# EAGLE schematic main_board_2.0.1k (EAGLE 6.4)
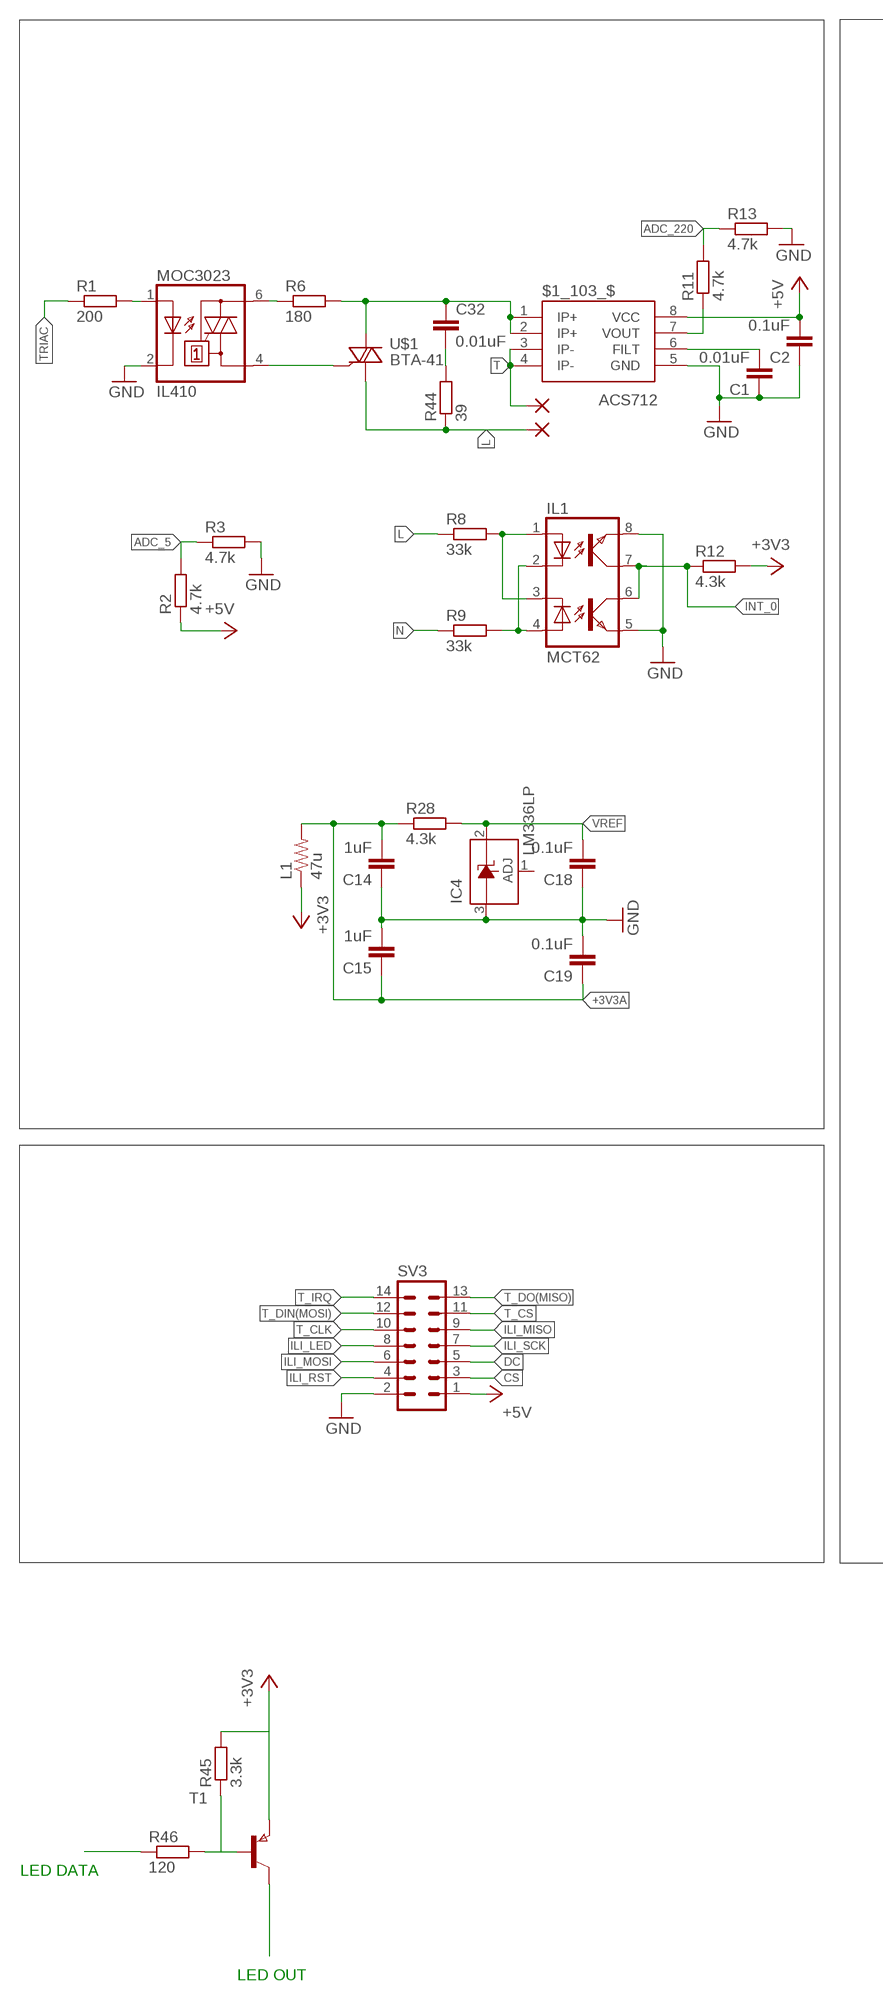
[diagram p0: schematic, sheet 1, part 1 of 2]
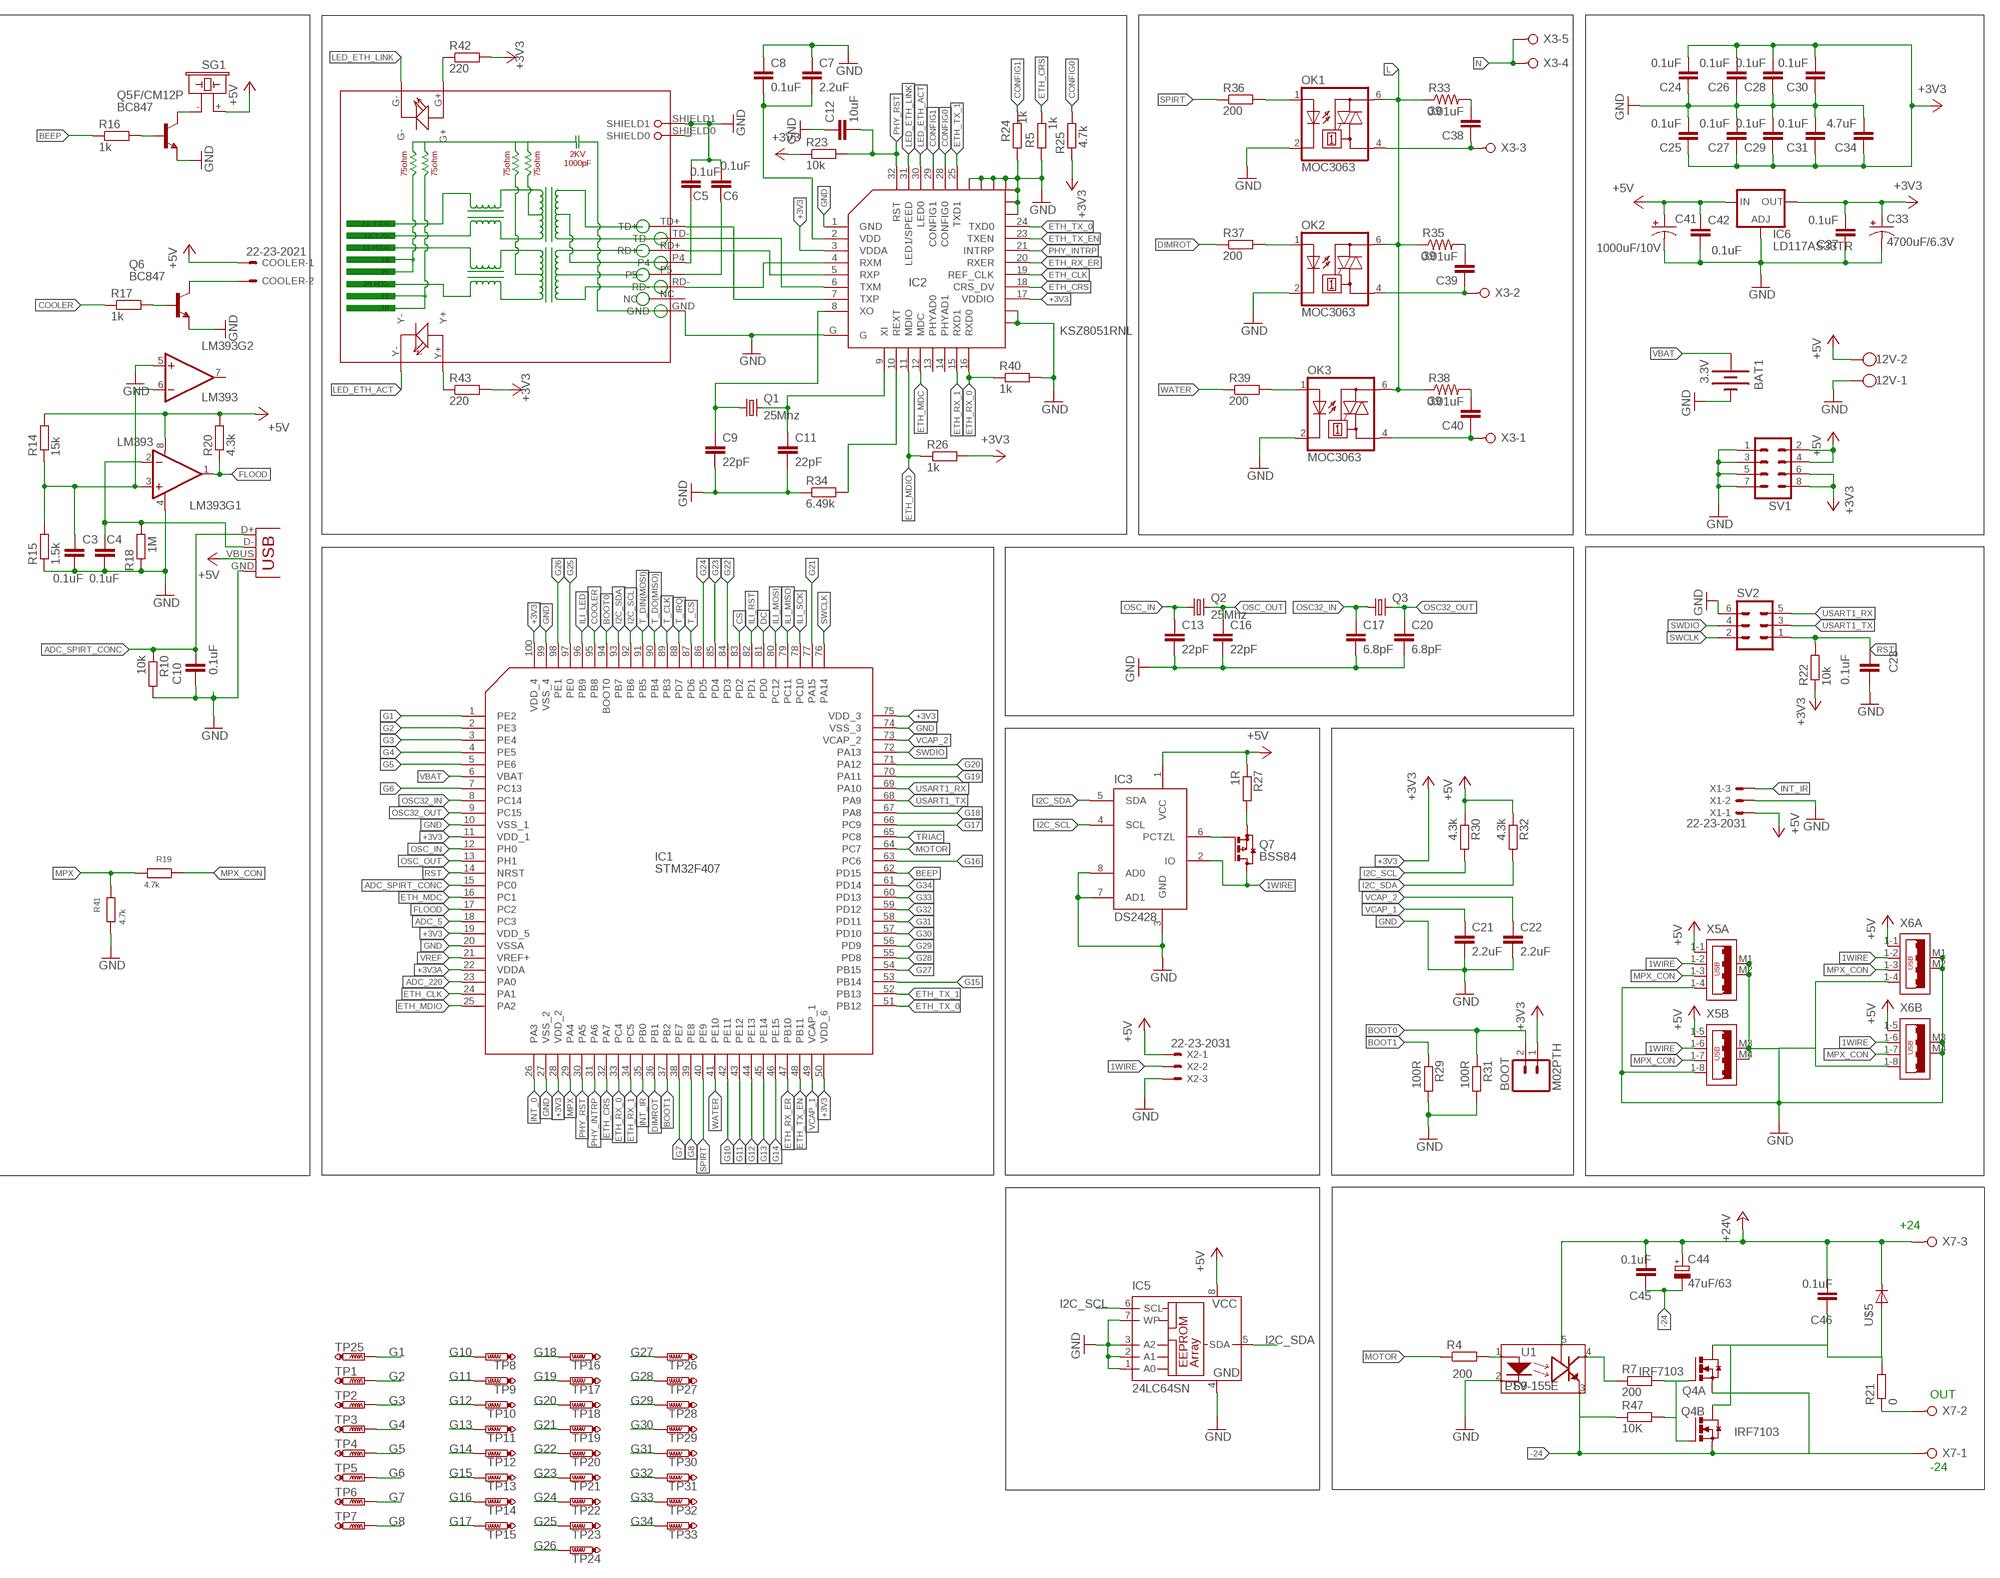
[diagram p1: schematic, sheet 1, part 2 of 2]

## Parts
12V  W237-102  [W237-102]
$1_103_$  ACS712  [SO08]
BAT1  3.3V  BATTERY20PTH  [BATTCOM_20MM_PTH]
BOOT  M02PTH  [1X02]
C1  0.01uF  C-EUC0603  [C0603]
C2  0.1uF  C-EUC0603  [C0603]
C3  0.1uF  C-EUC0603  [C0603]
C4  0.1uF  C-EUC0603  [C0603]
C5  0.1uF  C-EUC0603  [C0603]
C6  0.1uF  C-EUC0603  [C0603]
C7  2.2uF  C-EUC0603  [C0603]
C8  0.1uF  C-EUC0603  [C0603]
C9  22pF  C-EUC0603  [C0603]
C10  0.1uF  C-EUC0603  [C0603]
C11  22pF  C-EUC0603  [C0603]
C12  10uF  CAP1206  [1206]
C13  22pF  C-EUC0603  [C0603]
C14  1uF  C-EUC0603  [C0603]
C15  1uF  C-EUC0603  [C0603]
C16  22pF  C-EUC0603  [C0603]
C17  6.8pF  C-EUC0603  [C0603]
C18  0.1uF  C-EUC0603  [C0603]
C19  0.1uF  C-EUC0603  [C0603]
C20  6.8pF  C-EUC0603  [C0603]
C21  2.2uF  C-EUC0603  [C0603]
C22  2.2uF  C-EUC0603  [C0603]
C23  0.1uF  C-EUC0603  [C0603]
C24  0.1uF  C-EUC0603  [C0603]
C25  0.1uF  C-EUC0603  [C0603]
C26  0.1uF  C-EUC0603  [C0603]
C27  0.1uF  C-EUC0603  [C0603]
C28  0.1uF  C-EUC0603  [C0603]
C29  0.1uF  C-EUC0603  [C0603]
C30  0.1uF  C-EUC0603  [C0603]
C31  0.1uF  C-EUC0603  [C0603]
C32  0.01uF  C-EU075-032X103  [C075-032X103]
C33  4700uF/6.3V  CPOL-USE5-13  [E5-13]
C34  4.7uF  C-EUC0603  [C0603]
C37  0.1uF  C-EUC0603  [C0603]
C38  0.01uF  CAPPTH3  [CAP-PTH-LARGE]
C39  0.01uF  CAPPTH3  [CAP-PTH-LARGE]
C40  0.01uF  CAPPTH3  [CAP-PTH-LARGE]
C41  1000uF/10V  CPOL-USE5-8.5  [E5-8,5]
C42  0.1uF  C-EUC0603  [C0603]
C44  47uF/63  CPOL-EUE5-10.5  [E5-10,5]
C45  0.1uF  C-EUC0603  [C0603]
C46  0.1uF  C-EUC0603  [C0603]
COOLER  22-23-2021  [22-23-2021]
IC1  STM32F407  [LQFP100]
IC2  KSZ8051RNL  [QFN32]
IC3  DS2428  [SO08]
IC4  LM336LP  [TO92]
IC5  24LC64SN  [SO-08]
IC6  LD117AS33TR  [SOT223]
IL1  MCT62  [DIL8]
JP1  USB-B  USBPTH  [USB-B-PTH]
L  PAD-220  [PAD-220]
L1  47u  RESISTOR2010  [R2010]
LM393  LM393  [SO08]
MOC3023  IL410  [DIL06]
OK1  MOC3063  MOC3023M  [DIL06]
OK2  MOC3063  MOC3023M  [DIL06]
OK3  MOC3063  MOC3023M  [DIL06]
Q1  25Mhz  CRYSTALHC49U-V  [HC49U-V]
Q2  25Mhz  CRYSTALHC49U-V  [HC49U-V]
Q3  CRYSTALTC38H  [TC38H]
Q4  IRF7103  IRF8313P  [SO-08]
Q5  BC847  [SOT23]
Q6  BC847  [SOT23]
Q7  BSS84  [SOT23]
R1  200  R-EU_R0603  [R0603]
R2  4.7k  R-EU_R0603  [R0603]
R3  4.7k  R-EU_R0603  [R0603]
R4  200  R-EU_R0603  [R0603]
R5  1k  R-EU_R0603  [R0603]
R6  180  R-EU_0204/2V  [0204V]
R7  200  R-EU_R0603  [R0603]
R8  33k  R-EU_0617/5V  [0617V]
R9  33k  R-EU_0617/5V  [0617V]
R10  10k  R-EU_R0603  [R0603]
R11  4.7k  R-EU_R0603  [R0603]
R12  4.3k  R-EU_R0603  [R0603]
R13  4.7k  R-EU_R0603  [R0603]
R14  15k  R-EU_R0603  [R0603]
R15  1.5k  R-EU_R0603  [R0603]
R16  1k  R-EU_R0603  [R0603]
R17  1k  R-EU_R0603  [R0603]
R18  1M  R-EU_R0603  [R0603]
R19  4.7k  R-EU_R0603  [R0603]
R20  4.3k  R-EU_R0603  [R0603]
R21  0  R-EU_R1206  [R1206]
R22  10k  R-EU_R0603  [R0603]
R23  10k  R-EU_R0603  [R0603]
R24  1k  R-EU_R0603  [R0603]
R25  4.7k  R-EU_R0603  [R0603]
R26  1k  R-EU_R0603  [R0603]
R27  1R  R-EU_R0603  [R0603]
R28  4.3k  R-EU_R0603  [R0603]
R29  100R  R-EU_R0603  [R0603]
R30  4.3k  R-EU_R0603  [R0603]
R31  100R  R-EU_R0603  [R0603]
R32  4.3k  R-EU_R0603  [R0603]
R33  39  RESISTOR2512  [R2512]
R34  6.49k  R-EU_R0805  [R0805]
R35  39  RESISTOR2512  [R2512]
R36  200  R-EU_R0603  [R0603]
R37  200  R-EU_R0603  [R0603]
R38  39  RESISTOR2512  [R2512]
R39  200  R-EU_R0603  [R0603]
R40  1k  R-EU_R0603  [R0603]
R41  4.7k  R-EU_R0603  [R0603]
R42  220  R-EU_R0603  [R0603]
R43  220  R-EU_R0603  [R0603]
R44  39  R-EU_0613/5V  [P0613V]
R45  3.3k  R-EU_R0603  [R0603]
R46  120  R-EU_R0603  [R0603]
R47  10K  R-EU_R0603  [R0603]
RJ1  HR911105A  [HR911105A]
SG1  F/CM12P  [F/CM12P]
SV1  MA04-2  [MA04-2]
SV2  MA03-2  [MA03-2]
SV3  ML14  [ML14]
T  PAD-220  [PAD-220]
T1  PNPSOT23  [SOT-23]
TP1  PTR1MY0012X0024  [MY]
TP2  PTR1MY0012X0024  [MY]
TP3  PTR1MY0012X0024  [MY]
TP4  PTR1MY0012X0024  [MY]
TP5  PTR1MY0012X0024  [MY]
TP6  PTR1MY0012X0024  [MY]
TP7  PTR1MY0012X0024  [MY]
TP8  PTR1MY0012X0024  [MY]
TP9  PTR1MY0012X0024  [MY]
TP10  PTR1MY0012X0024  [MY]
TP11  PTR1MY0012X0024  [MY]
TP12  PTR1MY0012X0024  [MY]
TP13  PTR1MY0012X0024  [MY]
TP14  PTR1MY0012X0024  [MY]
TP15  PTR1MY0012X0024  [MY]
TP16  PTR1MY0012X0024  [MY]
TP17  PTR1MY0012X0024  [MY]
TP18  PTR1MY0012X0024  [MY]
TP19  PTR1MY0012X0024  [MY]
TP20  PTR1MY0012X0024  [MY]
TP21  PTR1MY0012X0024  [MY]
TP22  PTR1MY0012X0024  [MY]
TP23  PTR1MY0012X0024  [MY]
TP24  PTR1MY0012X0024  [MY]
TP25  PTR1MY0012X0024  [MY]
TP26  PTR1MY0012X0024  [MY]
TP27  PTR1MY0012X0024  [MY]
TP28  PTR1MY0012X0024  [MY]
TP29  PTR1MY0012X0024  [MY]
TP30  PTR1MY0012X0024  [MY]
TP31  PTR1MY0012X0024  [MY]
TP32  PTR1MY0012X0024  [MY]
TP33  PTR1MY0012X0024  [MY]
U1  LTV-155E  OPTO:PS9__  [PANASONIC_SOP5]
U$1  BTA-41  [TOP3L]
U$5  DIODE-SMB  [SMB]
X1  22-23-2031  [22-23-2031]
X2  22-23-2031  [22-23-2031]
X3  W237-05P  [W237-5P]
X5  USB_3PSHIELD-85-32003-00X-1  [85-32003-00X-1]
X6  USB_3PSHIELD-85-32003-00X-1  [85-32003-00X-1]
X7  W237-03P  [W237-133]

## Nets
1WIRE: IC3.2(IO) Q7.3(D) X2.2 X5.1-2 X5.1-6 X6.1-2 X6.1-6
+3V3 [+3V3]: BOOT.1 C24.2 C25.1 C26.2 C27.1 C28.2 C29.1 C30.2 C31.1 C33.+ C34.1 C37.2 IC1.11(VDD_1) IC1.19(VDD_5) IC1.28(VDD_2) IC1.50(VDD_6) IC1.75(VDD_3) IC1.100(VDD_4) IC2.3(VDDA) IC2.17(VDDIO) IC6.4(OUT) L1.1 R12.2 R22.1 R23.1 R25.1 R26.2 R42.2 R43.2 R45.2 SV1.6 SV1.8 T1.2(E)
+3V3A: C14.2 C15.1 C19.1 IC1.22(VDDA) L1.2 R28.1
+5V [+5V]: 12V.2 $1_103_$.8(VCC) C2.2 C41.+ C42.2 COOLER.1 IC3.1(VCC) IC5.8(VCC) IC6.3(IN) JP1.VBUS LM393.8(V+) R2.1 R14.2 R20.2 R27.1 R30.1 R32.1 SG1.+ SV1.2 SV1.4 SV3.1 X1.1 X2.1 X5.1-1 X5.1-5 X6.1-1 X6.1-5
+24V: C44.+ C45.2 C46.2 U1.5(VCC) U$5.C X7.3
-24: C44.- C45.1 Q4.1(B:S) Q4.3(A:S) R47.1 U1.3(COM) X7.1
ADC_5: IC1.18(PC3) R2.2 R3.1
ADC_220: IC1.23(PA0) R11.2 R13.1
ADC_SPIRT_CONC: C10.2 IC1.15(PC0) JP1.D+ R10.1
BEEP: IC1.62(PD15) R16.1
BOOT0: BOOT.2 IC1.94(BOOT0) R31.1
BOOT1: IC1.37(PB2) R29.1
CONFIG0: IC2.28(CONFIG0) R25.2
CONFIG1: IC2.29(CONFIG1) R24.2
COOLER: IC1.95(PB8) R17.1
CS: IC1.83(PD2) SV3.3
DC: IC1.81(PD0) SV3.5
DIMROT: IC1.36(PB1) R37.1
DRAIN: C46.1 Q4.5(A:D) Q4.6(A:D) Q4.7(B:D) Q4.8(B:D) R21.2 U$5.A
ETH_CLK: IC1.24(PA1) IC2.19(REF_CLK)
ETH_CRS: IC1.32(PA7) IC2.18(CRS_DV) R5.2
ETH_MDC: IC1.16(PC1) IC2.12(MDC)
ETH_MDIO: IC1.25(PA2) IC2.11(MDIO) R26.1
ETH_RX_0: IC1.33(PC4) IC2.16(RXD0) R40.1
ETH_RX_1: IC1.34(PC5) IC2.15(RXD1)
ETH_RX_ER: IC1.47(PB10) IC2.20(RXER)
ETH_TX_0: IC1.51(PB12) IC2.24(TXD0)
ETH_TX_1: IC1.52(PB13) IC2.25(TXD1)
ETH_TX_EN: IC1.48(PB11) IC2.23(TXEN)
FLOOD: IC1.17(PC2) LM393.1(OUT) R20.1
G1: IC1.1(PE2) TP25.P$1(TP)
G2: IC1.2(PE3) TP1.P$1(TP)
G3: IC1.3(PE4) TP2.P$1(TP)
G4: IC1.4(PE5) TP3.P$1(TP)
G5: IC1.5(PE6) TP4.P$1(TP)
G6: IC1.7(PC13) TP5.P$1(TP)
G7: IC1.38(PE7) TP6.P$1(TP)
G8: IC1.39(PE8) TP7.P$1(TP)
G10: IC1.42(PE11) TP8.P$1(TP)
G11: IC1.43(PE12) TP9.P$1(TP)
G12: IC1.44(PE13) TP10.P$1(TP)
G13: IC1.45(PE14) TP11.P$1(TP)
G14: IC1.46(PE15) TP12.P$1(TP)
G15: IC1.53(PB14) TP13.P$1(TP)
G16: IC1.63(PC6) TP14.P$1(TP)
G17: IC1.66(PC9) TP15.P$1(TP)
G18: IC1.67(PA8) TP16.P$1(TP)
G19: IC1.70(PA11) TP17.P$1(TP)
G20: IC1.71(PA12) TP18.P$1(TP)
G21: IC1.77(PA15) TP19.P$1(TP)
G22: IC1.84(PD3) TP20.P$1(TP)
G23: IC1.85(PD4) TP21.P$1(TP)
G24: IC1.86(PD5) TP22.P$1(TP)
G25: IC1.97(PE0) TP23.P$1(TP)
G26: IC1.98(PE1) TP24.P$1(TP)
G27: IC1.54(PB15) TP26.P$1(TP)
G28: IC1.55(PD8) TP27.P$1(TP)
G29: IC1.56(PD9) TP28.P$1(TP)
G30: IC1.57(PD10) TP29.P$1(TP)
G31: IC1.58(PD11) TP30.P$1(TP)
G32: IC1.59(PD12) TP31.P$1(TP)
G33: IC1.60(PD13) TP32.P$1(TP)
G34: IC1.61(PD14) TP33.P$1(TP)
GND: 12V.1 $1_103_$.5(GND) BAT1.2(-) C1.1 C2.1 C3.1 C4.1 C5.2 C6.2 C7.1 C8.1 C9.2 C10.1 C11.2 C12.1 C13.2 C14.1 C15.2 C16.2 C17.2 C18.1 C19.2 C20.2 C21.2 C22.2 C23.2 C24.1 C25.2 C26.1 C27.2 C28.1 C29.2 C30.1 C31.2 C33.- C34.2 C37.1 C41.- C42.1 IC1.10(VSS_1) IC1.20(VSSA) IC1.27(VSS_2) IC1.74(VSS_3) IC1.99(VSS_4) IC2.1(GND) IC2.G IC2.P$2(GND1) IC2.P$3(GND2) IC2.P$4(GND3) IC2.P$5(GND4) IC2.P$6(GND5) IC2.P$7(GND6) IC2.P$8(GND7) IC2.P$9(GND8) IC2.P$10(GND9) IC3.3(GND) IC3.7(AD1) IC3.8(AD0) IC4.3(A) IC5.1(A0) IC5.2(A1) IC5.3(A2) IC5.4(GND) IC5.7(WP) IC6.1(ADJ) IL1.5(EMIT1) IL1.8(EMIT) JP1.GND LM393.4(V-) LM393.5(+IN) MOC3023.2(C) OK1.2(C) OK2.2(C) OK3.2(C) Q5.2(E) Q6.2(E) R3.2 R5.1 R10.2 R13.2 R15.1 R18.1 R24.1 R29.2 R31.2 R34.1 R40.2 R41.2 RJ1.GND RJ1.SHIELD0 RJ1.SHIELD1 SV1.1 SV1.3 SV1.5 SV1.7 SV2.6 SV3.2 U1.2(K) X1.2 X2.3 X5.1-4 X5.1-8 X5.M1(A:M6) X5.M2(A:M7) X5.M3(B:M6) X5.M4(B:M7) X6.1-4 X6.1-8 X6.M1(A:M6) X6.M2(A:M7) X6.M3(B:M6) X6.M4(B:M7)
I2C_SCL: IC1.92(PB6) IC3.4(SCL) IC5.6(SCL) R30.2
I2C_SDA: IC1.93(PB7) IC3.5(SDA) IC5.5(SDA) R32.2
ILI_LED: IC1.96(PB9) SV3.8
ILI_MISO: IC1.79(PC11) SV3.9
ILI_MOSI: IC1.80(PC12) SV3.6
ILI_RST: IC1.82(PD1) SV3.4
ILI_SCK: IC1.78(PC10) SV3.7
INT_0: IC1.26(PA3) IL1.6(COL1) IL1.7(COL) R12.1
INT_IR: IC1.35(PB0) X1.3
L: L.1(P) OK1.6(A2) OK2.6(A2) OK3.6(A2) R8.1 R33.1 R35.1 R38.1 R44.1 U$1.A1
LED_ETH_ACT: IC2.30(LED0) RJ1.Y-
LED_ETH_LINK: IC2.31(LED1/SPEED) RJ1.G-
LT: $1_103_$.1(IP+) $1_103_$.2(IP+) C32.1 R6.2 U$1.A2
MOTOR: IC1.64(PC7) R4.1
MPX: IC1.29(PA4) R19.2 R41.1
MPX_CON: R19.1 X5.1-3 X5.1-7 X6.1-3 X6.1-7
N: R9.1 X3.4 X3.5
N$1: IC3.6(PCTZL) Q7.1(G)
N$2: Q5.3(C) SG1.-
N$3: Q5.1(B) R16.2
N$4: COOLER.2 Q6.3(C)
N$5: Q6.1(B) R17.2
N$6: IC2.10(REXT) R34.2
N$7: R4.2 U1.1(A)
N$8: C7.2 C8.2 IC2.2(VDD)
N$9: C9.1 IC2.8(XO) Q1.1
N$10: C11.1 IC2.9(XI) Q1.2
N$11: IC2.5(RXP) RJ1.RD+
N$12: IC2.6(TXM) RJ1.TD-
N$13: IC2.7(TXP) RJ1.TD+
N$14: C5.1 RJ1.P4
N$15: IC2.4(RXM) RJ1.RD-
N$16: C6.1 RJ1.P5
N$17: IL1.1(A) IL1.3(C1) R8.2
N$18: Q4.2(B:G) Q4.4(A:G) R7.2 R47.2
N$19: T1.1(C)
N$21: C32.2 R44.2
N$22: R42.1 RJ1.G+
N$23: C3.2 LM393.3(+IN) LM393.6(-IN) R14.1 R15.2
N$24: C4.2 JP1.D- LM393.2(-IN) R18.2
N$26: Q7.2(S) R27.2
N$27: R45.1 R46.2 T1.3(B)
N$28: R7.1 U1.4(OC)
N$29: OK1.1(A) R36.2
N$30: OK2.1(A) R37.2
N$31: MOC3023.6(A2) R6.1
N$32: $1_103_$.7(VOUT) R11.1
N$33: IL1.2(C) IL1.4(A1) R9.2
N$34: C39.2 R35.2
N$35: MOC3023.1(A) R1.2
N$36: $1_103_$.6(FILT) C1.2
N$37: C38.2 R33.2
N$38: R21.1 X7.2
N$39: R43.1 RJ1.Y+
N$40: R46.1
N$42: C38.1 OK1.4(A1) X3.3
N$43: C39.1 OK2.4(A1) X3.2
N$44: OK3.1(A) R39.2
N$45: C40.2 R38.2
N$48: C40.1 OK3.4(A1) X3.1
OSC32_IN: C17.1 IC1.8(PC14) Q3.1
OSC32_OUT: C20.1 IC1.9(PC15) Q3.2
OSC_IN: C13.1 IC1.12(PH0) Q2.1
OSC_OUT: C16.1 IC1.13(PH1) Q2.2
PHY_INTRP: IC1.31(PA6) IC2.21(INTRP)
PHY_RST: C12.2 IC1.30(PA5) IC2.32(RST) R23.2
RST: C23.1 IC1.14(NRST) R22.2 SV2.1
SPIRT: IC1.40(PE9) R36.1
SWCLK: IC1.76(PA14) SV2.2
SWDIO: IC1.72(PA13) SV2.4
T: $1_103_$.3(IP-) $1_103_$.4(IP-) T.1(P)
T_CLK: IC1.89(PB3) SV3.10
T_CS: IC1.87(PD6) SV3.11
T_DIN(MOSI): IC1.91(PB5) SV3.12
T_DO(MISO): IC1.90(PB4) SV3.13
T_IRQ: IC1.88(PD7) SV3.14
TRIAC: IC1.65(PC8) R1.1
TRIAC_V: MOC3023.4(A1) U$1.G3(G)
USART1_RX: IC1.69(PA10) SV2.5
USART1_TX: IC1.68(PA9) SV2.3
VBAT: BAT1.1(+) IC1.6(VBAT)
VCAP_1: C21.1 IC1.49(VCAP_1)
VCAP_2: C22.1 IC1.73(VCAP_2)
VREF: C18.2 IC1.21(VREF+) IC4.2(C) R28.2
WATER: IC1.41(PE10) R39.1
Unconnected: IC2.13(PHYAD0) IC2.14(PHYAD1) IC4.1(ADJ) LM393.7(OUT) RJ1.NC

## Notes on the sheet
- +24
- OUT
- LED DATA
- -24
- LED OUT

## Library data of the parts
12V = con-wago-500:W237-102: WAGO SCREW CLAMP; MPN: 237-102; OC_FARNELL: unknown; OC_NEWARK: 70K9898
$1_103_$ = SparkFun:ACS712
BAT1 = SparkFun:BATTERY: Battery Holders
BOOT = SparkFun-Connectors:M02: Standard 2-pin 0.1" header. Use with
C1-C11 C13-C31 C34 C37 C42 C45 C46 = rcl:C-EU: CAPACITOR, European symbol
C12 C38-C40 = SparkFun:CAP: Capacitor
C32 = resistor:C-EU: CAPACITOR, European symbol
C33 C41 = resistor:CPOL-US: POLARIZED CAPACITOR, American symbol
C44 = resistor:CPOL-EU: POLARIZED CAPACITOR, European symbol
COOLER = con-molex:22-23-2021: .100" (2.54mm) Center Header - 2 Pin; MF: MOLEX; MPN: 22-23-2021; OC_FARNELL: 1462926; OC_NEWARK: 25C3832
IC1 = upravliator:STM32F407
IC2 = upravliator:KSZ8051RNL
IC3 = upravliator:DS2428
IC4 = linear:LM336: 2.5-V INTEGRATED REFERENCE CIRCUITS LM236 Source: http://focus.ti.com/lit/ds/symlink/lm336-2.5.pdf
IC5 = microchip:24*: Serial EEPROM I2C; MF: MICROCHIP; MPN: 24LC64-I/SN; OC_FARNELL: 9758070; OC_NEWARK: 12C2020
IC6 = v-reg:LD117A?*: Low drop fixed and adjustable positive voltage regulators 1 A Source: http://www.st.com/stonline/products/literature/ds/7194/ld1117axx.pdf
IL1 = upravliator:MCT62
JP1 = SparkFun-Connectors:USB: USB Connectors USB-B-PTH is fully proven SKU : PRT-00139/CONN-08278 USB-miniB is fully proven SKU : PRT-00587 USB-A-PCB is untested. USB-A-H is throughly reviewed, but untested. Spark Fun Electronics SKU : PRT-00437 USB-B-SMT is throughly reviewed, but untested. Needs silkscreen touching up.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; PROD_ID: CONN-08278
L T = upravliator:PAD-220
L1 R33 R35 R38 = SparkFun:RESISTOR: Resistor
LM393 = SparkFun:LM393
MOC3023 = optocoupler:IL410: SIEMENS OPTO COUPLER; MF: VISHAY/TELEFUNKEN; MPN: IL410; OC_FARNELL: 1045434; OC_NEWARK: 58K1715
OK1-OK3 = optocoupler:MOC30*M: RANDOM-PHASE OPTOISOLATORS TRIAC DRIVER OUTPUT Source: http://www.fairchildsemi.com MOC3020-M.pdf; MF: FAIRCHILD SEMICONDUCTOR; MPN: MOC3023-M; OC_FARNELL: 1021367; OC_NEWARK: 72K8896
Q1 Q2 = crystal:CRYSTAL: CRYSTAL; OC_FARNELL: 1666969; OC_NEWARK: unknown
Q3 = SparkFun:CRYSTAL: Crystals
Q4 = transistor-power:IRF8313P: HEXFET(R) Power MOSFET Source: Data sheet
Q5 Q6 = transistor:BC847: NPN TRANSISTOR
Q7 = transistor-small-signal:BSS84: P-CHANNEL MOS FET
R1-R5 R10-R20 R22-R32 R34 R36 R37 R39-R43 R45 R46 = rcl:R-EU_: RESISTOR, European symbol
R6-R9 R21 R44 R47 = resistor:R-EU_: RESISTOR, European symbol
RJ1 = CONNECTER:HR911105A
SG1 = buzzer:F/CM12P: BUZZER; OC_FARNELL: unknown; OC_NEWARK: unknown
SV1 = con-lstb:MA04-2: PIN HEADER; OC_FARNELL: unknown; OC_NEWARK: unknown
SV2 = con-lstb:MA03-2: PIN HEADER; OC_FARNELL: unknown; OC_NEWARK: unknown
SV3 = con-harting-ml:ML14: HARTING; OC_FARNELL: unknown; OC_NEWARK: unknown
T1 = zetex:PNPSOT23: PNP TRANSISTOR; MPN: DSS20200L-7; OC_FARNELL: unknown; OC_NEWARK: 25R4554
TP1-TP33 = testpad:PTR1: TEST PIN
U1 = QuantumOptics:OPTO:PS9__: PS9xxx, Panasonic, 5-pin SMT optocouplers. Based on PS9121, http://www.cel.com/pdf/datasheets/ps9121.pdf.
U$1 = upravliator:BTA-41
U$5 = diode:DIODE-: DIODE
X1 X2 = con-molex:22-23-2031: .100" (2.54mm) Center Header - 3 Pin; MF: MOLEX; MPN: 22-23-2031; OC_FARNELL: 1462950; OC_NEWARK: 30C0862
X3 = con-wago-508:W237-05P: WAGO SREW CLAMP; OC_FARNELL: unknown; OC_NEWARK: unknown
X5 X6 = upravliator:USB_3PSHIELD-: Triple USB Connector Source: www.cypressindustries.com; OC_FARNELL: unknown; OC_NEWARK: unknown
X7 = con-wago-508:W237-03P: WAGO SREW CLAMP; OC_FARNELL: unknown; OC_NEWARK: unknown

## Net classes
0 default: width 0.203 mm, drill 0.203 mm, clearance 0.152 mm
1 GND: width 0.203 mm, drill 0.203 mm, clearance 0.152 mm to class 0
2 +3V3: width 0.254 mm, drill 0.203 mm, clearance 0.152 mm to class 0, clearance 0.152 mm to class 1
3 +5V: width 0.406 mm, drill 0.152 mm, clearance 0.203 mm to class 0, clearance 0.203 mm to class 1, clearance 0.203 mm to class 2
